ORGANIZATION_BLOCK OB 1
BEGIN
	// Test parsing of convenience operators.
	// Convenience operators are certain operators with missing white space.

	OPN	DB1
	OPN	DI1

	SET
	=	I0.1
	=	Q0.1
	=	M0.1
	=	L0.1
	=	DBX0.0
	=	DIX0.0

	L	100
	T	IB0
	T	IW0
	T	ID0
	T	QB0
	T	QW0
	T	QD0
	T	LB0
	T	LW0
	T	LD0
	T	MB0
	T	MW0
	T	MD0
	T	DBB0
	T	DBW0
	T	DBD0
	T	DIB0
	T	DIW0
	T	DID0

	A	T0
	=	M0.0
	A	C0
	=	M0.0


	CALL SFC 46 // STOP CPU
END_ORGANIZATION_BLOCK


DATA_BLOCK DB 1
STRUCT
	VARIABLE : DWORD
END_STRUCT
BEGIN
	VARIABLE := DW#16#1
END_DATA_BLOCK
